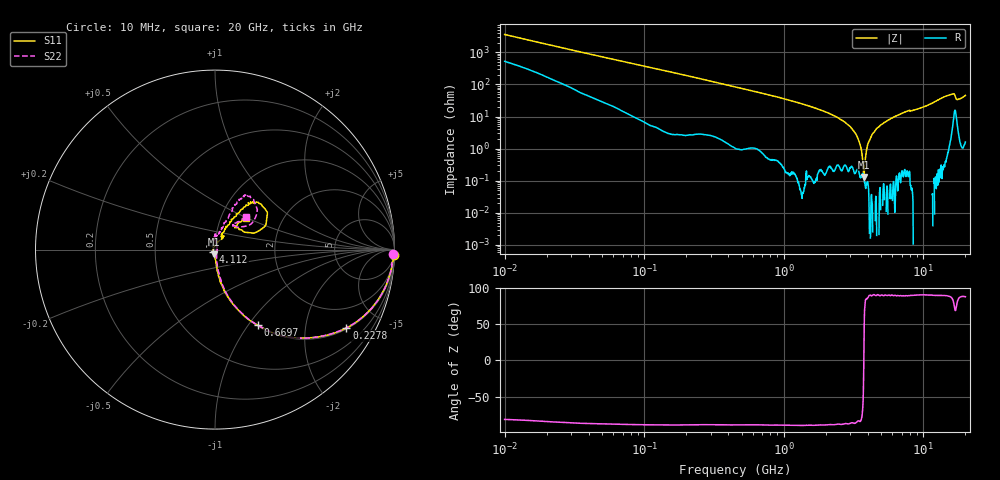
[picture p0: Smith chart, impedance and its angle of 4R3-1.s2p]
!Keysight Technologies,P5008B,MY61100088,A.16.20.02
!Date: Monday, May 27, 2024 15:28:16
!Correction: S11(C* 2-Port  )
!S21(C* 2-Port  )
!S12(C* 2-Port  )
!S22(C* 2-Port  )
!S2P File: Measurements: S11, S21, S12, S22:Log Frequency Sweep
# Hz S  dB  R 50
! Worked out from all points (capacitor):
!   1601 points, 10 MHz to 20 GHz, reference 50 ohm
!   read as one part in series: C = 4.47 pF near 10.39 MHz
!   lowest |Z| = 131 mohm at 3.757 GHz (marker M1)
!   series resonance near 3.745 GHz, so ESL is about 400 pH
!   S11 on the Smith chart (normalised r, x): 10 MHz: 6, -72; 227.8 MHz: 1.04, -3.33; 669.7 MHz: 1.01, -1.12; 4.112 GHz: 0.98, -0.02; 20 GHz: 1.32, +0.49
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1e7  -0.02 -1.6  -31.18 80.1  -31.20 80.1  -0.05 -1.6
3.555162e7  -0.09 -5.6  -20.18 81.4  -20.19 81.4  -0.09 -5.6
1.263918e8  -0.52 -18.6  -9.96 70.6  -9.97 70.6  -0.51 -18.6
2.277973e8  -1.39 -30.8  -5.87 58.3  -5.88 58.3  -1.39 -30.7
4.472136e8  -3.86 -49.7  -2.40 39.7  -2.41 39.7  -3.85 -49.6
6.69703e8  -6.28 -60.4  -1.23 28.7  -1.24 28.7  -6.28 -60.5
1.589917e9  -13.96 -79.3  -0.18 10.8  -0.19 10.8  -13.89 -78.0
2.70674e9  -21.41 -84.6  -0.03 3.1  -0.04 3.1  -21.35 -81.3
3.273198e9  -25.79 -89.8  -0.00 0.5  -0.01 0.5  -26.35 -79.7
3.756673e9  -31.77 -102.8  0.01 -1.4  -0.00 -1.4  -33.00 -63.2
4.111527e9  -36.36 -132.7  0.01 -2.6  -0.00 -2.6  -37.82 -31.6
4.457348e9  -39.33 -179.9  0.01 -3.8  0.00 -3.8  -38.99 14.7
5.652411e9  -29.10 80.0  0.01 -7.2  0.00 -7.2  -29.25 83.1
6.335038e9  -25.56 66.0  0.02 -9.0  0.00 -8.9  -25.97 88.0
7.588373e9  -21.60 57.0  -0.00 -12.1  -0.01 -12.1  -21.91 90.2
8.344716e9  -22.53 57.4  0.01 -13.7  0.01 -13.7  -22.64 88.1
9.854205e9  -21.02 67.4  0.01 -17.4  0.00 -17.5  -21.04 76.9
1.489756e10  -9.58 51.9  -0.49 -31.0  -0.50 -31.0  -9.55 61.8
1.630478e10  -8.89 39.8  -1.02 -34.2  -1.03 -34.2  -9.07 52.1
1.717946e10  -13.24 25.6  -0.96 -27.4  -0.97 -27.4  -14.21 40.7
1.792989e10  -15.23 44.5  -0.28 -30.6  -0.29 -30.6  -15.36 53.9
2e10  -12.17 45.1  -0.34 -39.1  -0.35 -39.1  -12.05 46.9
